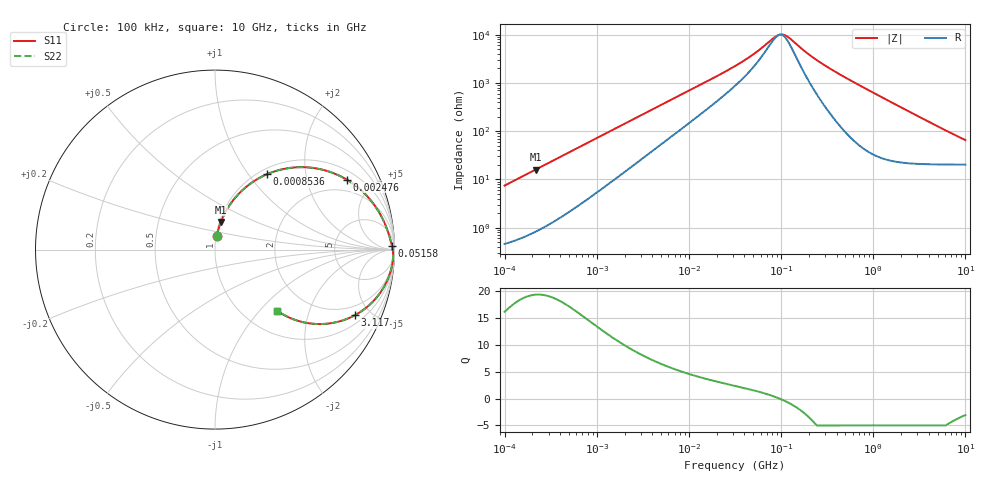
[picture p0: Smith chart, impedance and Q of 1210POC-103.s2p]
# MHz S MA R 50
!Freq  MagS11  AngS11  MagS21  AngS21  MagS12  AngS12  MagS22  AngS22
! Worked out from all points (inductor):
!   801 points, 100 kHz to 10 GHz, reference 50 ohm
!   read as one part in series: L = 11.8 uH near 105.9 kHz
!   highest Q = 19.4 at 217.5 kHz (marker M1), where L = 11.7 uH
!   self-resonance near 96.26 MHz
!   S11 on the Smith chart (normalised r, x): 100 kHz: 1.01, +0.15; 853.6 kHz: 1.09, +1.23; 2.476 MHz: 1.39, +3.49; 51.58 MHz: 47, +68; 3.117 GHz: 1.42, -4.01; 10 GHz: 1.41, -1.25
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0.1  0.07425 82.2  0.9927 -4.3  0.9927 -4.3  0.07425 82.2
0.2175204  0.1574 78.0  0.9794 -9.0  0.9794 -9.0  0.1574 78.0
0.4097321  0.2828 70.4  0.9437 -16.4  0.9437 -16.4  0.2828 70.4
0.6878599  0.4354 60.6  0.8726 -25.8  0.8726 -25.8  0.4354 60.6
0.8535913  0.5094 55.5  0.8257 -30.5  0.8257 -30.5  0.5094 55.5
1.433013  0.6873 41.8  0.6695 -43.2  0.6695 -43.2  0.6873 41.8
2.475996  0.8304 28.0  0.473 -55.6  0.473 -55.6  0.8304 28.0
4.663908  0.9188 16.2  0.2814 -65.3  0.2814 -65.3  0.9188 16.2
11.05987  0.9641 7.1  0.1266 -70.0  0.1266 -70.0  0.9641 7.1
31.62278  0.9822 2.3  0.04378 -64.8  0.04378 -64.8  0.9822 2.3
51.58222  0.9864 1.1  0.02404 -55.0  0.02404 -55.0  0.9864 1.1
85.35913  0.9895 0.2  0.01109 -19.0  0.01109 -19.0  0.9895 0.2
102.9201  0.9904 -0.1  0.009782 11.9  0.009782 11.9  0.9904 -0.1
122.3207  0.9912 -0.4  0.01147 39.4  0.01147 39.4  0.9912 -0.4
217.5204  0.9928 -1.6  0.02856 74.6  0.02856 74.6  0.9928 -1.6
459.727  0.992 -4.0  0.06999 81.4  0.06999 81.4  0.992 -4.0
841.3951  0.9845 -7.5  0.131 79.4  0.131 79.4  0.9845 -7.5
1474.857  0.9609 -13.0  0.2259 73.6  0.2259 73.6  0.9609 -13.0
2175.204  0.923 -18.6  0.3204 67.0  0.3204 67.0  0.923 -18.6
3117.095  0.8606 -25.2  0.4273 58.9  0.4273 58.9  0.8606 -25.2
5463.865  0.699 -36.4  0.6024 43.5  0.6024 43.5  0.699 -36.4
10000  0.4841 -44.5  0.7378 27.4  0.7378 27.4  0.4841 -44.5
